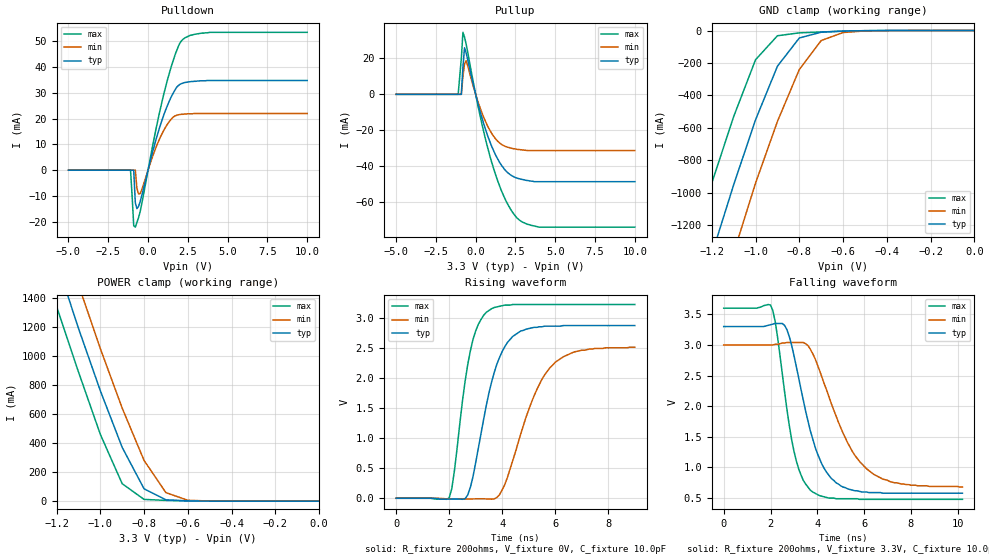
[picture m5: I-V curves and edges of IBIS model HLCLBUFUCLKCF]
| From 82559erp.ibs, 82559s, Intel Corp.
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[Model]   HLCLBUFUCLKCF
Model_type   I/O
Vinl  =   0.8V   | note : D101S spec
Vinh  =   2V   | note : D101S spec
|variable   typ   min  max
C_comp   2.96pF   NA   NA
| note : on die power/gnd supply distribution R/L/C
|   are not included in the simulation
|variable   typ   min   max
[Voltage range]   3.3V   3.0V   3.6V
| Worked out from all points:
|   slope of the pulldown table from 0 to 0.495 V, typ, clamps not added: 42 ohm
|   slope of the pullup table from 0 to 0.495 V, typ, clamps not added: 30.8 ohm
|   GND clamp passes 1 mA (typ) near -0.50 V on its own axis
|   POWER clamp passes 1 mA (typ) near -0.55 V on its own axis
|   rising waveform, R_fixture 200ohms, V_fixture 0V, C_fixture 10.0pF: 20-80 % time 867ps typ, 1.23ns min, 617ps max; typ from 0 V to 2.87 V
|   falling waveform, R_fixture 200ohms, V_fixture 3.3V, C_fixture 10.0pF: 20-80 % time 1.08ns typ, 1.57ns min, 752ps max; typ from 3.3 V to 0.58 V
| note : all DC corves are with 0.2 OHM res. series to the PAD.
[GND_clamp]
| Voltage  I(typ)   I(min)   I(max)
-5V       -19.9A     -20.3A     -19.5A
-1.3V     -1.83A     -2.26A     -1.39A
-1.2V     -1.38A     -1.81A     -940mA
-1.1V     -950mA     -1.37A     -530mA
-1V       -550mA     -940mA     -180mA
-900mV    -220mA     -560mA     -32.3mA
-800mV    -45.9mA    -240mA     -14.4mA
-700mV    -10.3mA    -61.7mA    -8.98mA
-600mV    -3.4mA     -12.4mA    -4.05mA
-500mV    -950uA     -2.36mA    -1.01mA
0V        0A         0A         0A
[PullDown]
|Voltage  I(typ)   I(min)   I(max)
-5V       0A         0A         0A
-1.1V     0A         0A         0A
-900mV    0A         0A         -21.5mA
-800mV    -12.6mA    0A         -22.1mA
-700mV    -14.9mA    -6.97mA    -20.3mA
-500mV    -12.3mA    -9.1mA     -16.2mA
500mV     11.9mA     8.83mA     16mA
1V        21.6mA     15.6mA     29.8mA
1.7V      31.2mA     21.1mA     44.8mA
2.1V      33.6mA     21.7mA     50.2mA
3.9V      34.8mA     22mA       53.5mA
10V       34.8mA     22mA       53.5mA
[POWER_clamp]
|Voltage  I(typ)   I(min)   I(max)
-5V       20.3A      20.5A      20A
-1.3V     2.11A      2.41A      1.81A
-1.2V     1.65A      1.94A      1.34A
-1.1V     1.19A      1.49A      890mA
-1V       760mA      1.05A      460mA
-900mV    370mA      640mA      120mA
-800mV    84.8mA     280mA      11.9mA
-700mV    8.82mA     58.3mA     4.9mA
-600mV    1.74mA     5.95mA     1.41mA
-500mV    290uA      690uA      150uA
0V        1.33nA     19.2nA     450pA
[PullUp]
|Voltage  I(typ)   I(min)   I(max)
-5V       0A         0A         0A
-1.1V     0A         0A         0A
-900mV    0A         0A         20mA
-800mV    15.2mA     10mA       34.5mA
-700mV    25.9mA     16.8mA     31.9mA
-600mV    23.1mA     18.7mA     28mA
200mV     -6.95mA    -5.52mA    -8.71mA
900mV     -26.5mA    -20.1mA    -34.5mA
1.7V      -40.4mA    -28.3mA    -55.3mA
2.5V      -46.3mA    -30.4mA    -67.8mA
4V        -48.6mA    -31.3mA    -73.9mA
10V       -48.6mA    -31.3mA    -73.9mA
[Ramp]
|Variable   typ   min   max
dV/dt_r   1.75/0.9n   1.49/1.2n   0.99/0.6n
dV/dt_f   1.69/1.1n   1.43/1.6n   1.73/0.7n
R_load  = 200ohms
[Rising Waveform]
|   note : pad parasitics are not incloded
R_fixture   = 200ohms
V_fixture   = 0V
C_fixture   = 10.0pF
|Time   typ(V)   min(V)   max(V)
0s        -17.95nV   52.29nV    -380pV
2ns       -13.19mV   -12.63mV   5.01mV
2.2ns     -12.37mV   -12.77mV   460mV
2.7ns     54.6mV     -10.99mV   2.22V
3ns       590mV      -10.02mV   2.78V
3.4ns     1.54V      -10.52mV   3.09V
4.2ns     2.59V      350mV      3.21V
5.1ns     2.83V      1.59V      3.22V
5.8ns     2.86V      2.17V      3.22V
9ns       2.87V      2.51V      3.22V
[Falling Waveform]
|   note : pad parasitics are not incloded
R_fixture   = 200ohms
V_fixture   = 3.3V
V_fixture_min   = 3.0V
V_fixture_max   = 3.6V
C_fixture   = 10.0pF
|Time   typ   min   max
0s        3.3V       3V         3.6V
2ns       3.33V      3V         3.65V
2.2ns     3.35V      3.01V      3.38V
2.7ns     3.25V      3.04V      1.95V
3.1ns     2.65V      3.04V      1.11V
3.7ns     1.6V       2.93V      630mV
4.6ns     820mV      2.04V      500mV
5.3ns     650mV      1.4V       490mV
6.1ns     600mV      980mV      480mV
10.2ns    580mV      680mV      480mV
